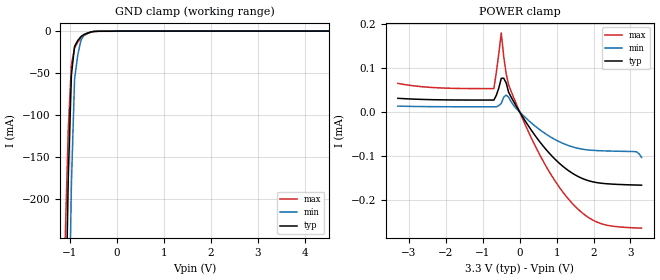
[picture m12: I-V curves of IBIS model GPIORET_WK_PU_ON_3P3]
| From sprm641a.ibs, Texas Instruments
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|   Model Cell GPIORET_WK_PU_ON_3P3
|GPIORET_WK_PU_ON_3P3
[Model]   GPIORET_WK_PU_ON_3P3
Model_type   Input
Polarity   Non-Inverting
Vinl =  0.8
Vinh =  2
C_comp   5.345208p   4.561426p   6.022817p
[Model Spec]
Vinl   0.8   0.8   0.8
Vinh   2   2   2
[Temperature Range]   25   155   -40
[Voltage Range]   3.3   2.97   3.63
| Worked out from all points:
|   GND clamp passes 1 mA (typ) near -0.54 V on its own axis
| Nom Voltages:
|   BIASFET=3.3, VDD=1.2, VDDS=3.3, VSS=0
| Min Voltages:
|   BIASFET=2.97, VDD=1.08, VDDS=2.97, VSS=0
| Max Voltages:
|   BIASFET=3.63, VDD=1.32, VDDS=3.63, VSS=0
[POWER_clamp]
|   voltage   I(typ)   I(min)   I(max)
-3.3V     31.22uA    13.5uA     64.95uA
-700mV    27.24uA    11.95uA    53.12uA
-500mV    76.46uA    19.77uA    179.4uA
-433.3mV  76.57uA    33.8uA     125.7uA
-366.7mV  65.99uA    38.44uA    86.4uA
-300mV    44.74uA    33.7uA     61.57uA
433.3mV   -55.14uA   -32.83uA   -78.95uA
1.1V      -118uA     -68.32uA   -173.5uA
1.567V    -145.3uA   -81.87uA   -219uA
2.033V    -159uA     -87.03uA   -246.9uA
3.167V    -165.3uA   -90.11uA   -262.6uA
3.3V      -165.6uA   -102.8uA   -263uA
[GND_clamp]
|   voltage   I(typ)   I(min)   I(max)
-3.3V     -16.36A    -15.08A    -17.18A
-1.1V     -382.1mA   -717.8mA   -250.1mA
-1.033V   -173.3mA   -402.2mA   -116.4mA
-966.7mV  -52.02mA   -182.1mA   -39.81mA
-900mV    -18.21mA   -57.44mA   -20.35mA
-833.3mV  -11.38mA   -28.89mA   -13.21mA
-766.7mV  -6.658mA   -11.29mA   -8.223mA
-700mV    -4.058mA   -4.616mA   -5.385mA
-500mV    -482.9uA   -556.9uA   -624.5uA
-33.33mV  0A         0A         0A
6.6V      0A         0A         0A
